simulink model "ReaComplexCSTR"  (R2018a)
settings: Solver=VariableStepAuto  StartTime=0.0  StopTime=10000  RelTol=1e-3
undefined symbols (not defined in the file): e729db96ecb7, f30486205ece, ReaComplexCSTR, sdiscope

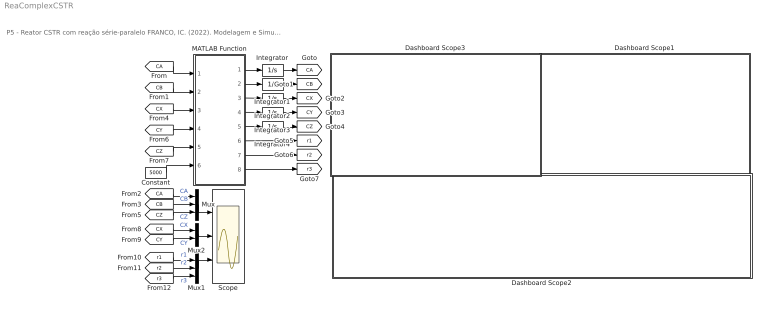
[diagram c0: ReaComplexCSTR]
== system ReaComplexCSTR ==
  note: P5 - Reator CSTR com reação série-paralelo FRANCO, IC. (2022). Modelagem e Simulação: Problemas Típicos da Engenharia Química para Simulação e Análise. NOTAS DE AULA INOVADORAS. The Journal of Engineering and Exact Sciences. Material Complementar.
  Constant : Constant  Value=5000
  Dashboard Scope1 : Subsystem  DialogController=hmiCreateDDGDialog  IsWebBlock=on  mask(MWDashboardBlock){webBlockId=67a52530-171f-4111-9f33-f30486205ece, webBlockType=sdiscope, ShowInitialText=on, HMISrcModelName=ReaComplexCSTR}
      mask prompts: webBlockId "WebBlock Id"; webBlockType "WebBlock Type"; HMISrcModelName "Source Model"
      mask help: SimulinkHMI:dialogs:HMIScopeDialogDesc
  Dashboard Scope2 : Subsystem  DialogController=hmiCreateDDGDialog  IsWebBlock=on  mask(MWDashboardBlock){webBlockId=01cdbba2-3691-40b7-94a4-e729db96ecb7, webBlockType=sdiscope, ShowInitialText=on, HMISrcModelName=ReaComplexCSTR}
      mask prompts: webBlockId "WebBlock Id"; webBlockType "WebBlock Type"; HMISrcModelName "Source Model"
      mask help: SimulinkHMI:dialogs:HMIScopeDialogDesc
  Dashboard Scope3 : Subsystem  DialogController=hmiCreateDDGDialog  IsWebBlock=on  mask(MWDashboardBlock){webBlockId=9a3adbde-0cc4-4c14-8736-21e25775a34c, webBlockType=sdiscope, ShowInitialText=on, HMISrcModelName=ReaComplexCSTR}
      mask prompts: webBlockId "WebBlock Id"; webBlockType "WebBlock Type"; HMISrcModelName "Source Model"
      mask help: SimulinkHMI:dialogs:HMIScopeDialogDesc
  Integrator : Integrator  InitialCondition=0.4
  Integrator1 : Integrator  InitialCondition=0.6
  Integrator2 : Integrator
  Integrator3 : Integrator
  Integrator4 : Integrator
  MATLAB Function : MATLAB Function  TreatAsAtomicUnit=on
  Mux : Mux  Inputs=3
  Mux1 : Mux  Inputs=3
  Mux2 : Mux  Inputs=2
  Scope : Scope  NumInputPorts=3
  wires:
  Integrator1/1 -> [CB]
  MATLAB Function/2(dCB) -> Integrator1/1
  [CB] -> MATLAB Function/2(CB)
  Integrator/1 -> [CA]
  [CA] -> MATLAB Function/1(CA)
  MATLAB Function/1(dCA) -> Integrator/1
  MATLAB Function/3(dCX) -> Integrator2/1
  Integrator2/1 -> [CX]
  MATLAB Function/5(dCZ) -> Integrator4/1
  MATLAB Function/4(dCY) -> Integrator3/1
  Integrator4/1 -> [CZ]
  Integrator3/1 -> [CY]
  MATLAB Function/6(r1) -> [r1]
  MATLAB Function/7(r2) -> [r2]
  MATLAB Function/8(r3) -> [r3]
  Constant/1 -> MATLAB Function/6(tau)
  [CX] -> MATLAB Function/3(CX)
  [CY] -> MATLAB Function/4(CY)
  [CZ] -> MATLAB Function/5(CZ)
  [CA] -> Mux/1  "CA"
  [CB] -> Mux/2  "CB"
  [r1] -> Mux1/1  "r1"
  [r2] -> Mux1/2  "r2"
  [r3] -> Mux1/3  "r3"
  [CX] -> Mux2/1  "CX"
  [CY] -> Mux2/2  "CY"
  Mux2/1 -> Scope/2
  Mux1/1 -> Scope/3
  Mux/1 -> Scope/1
  [CZ] -> Mux/3  "CZ"

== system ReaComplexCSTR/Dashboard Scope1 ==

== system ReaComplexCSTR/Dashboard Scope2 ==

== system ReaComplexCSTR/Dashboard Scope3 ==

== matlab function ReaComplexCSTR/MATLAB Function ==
function [dCA,dCB,dCX,dCY,dCZ,r1,r2,r3] = fcn(CA,CB,CX,CY,CZ,tau)
%% Parâmetros
CA0  = 0.4;
CB0  = 0.6;
CX0  = 0.0;
CY0  = 0.0;
CZ0  = 0.0;
k1   = 0.0005;
k2   = 0.0500;
k3   = 0.0200;

%% Equações auxiliares;
r1 = k1*CA*CB;
r2 = k2*CB*CX;
r3 = k3*CB*CY;

%% Modelo matemático
dCA = (1/tau)*(CA0-CA)-r1;
dCB = (1/tau)*(CB0-CB)-r1-r2-r3;
dCX = (1/tau)*(CX0-CX)+r1-r2;
dCY = (1/tau)*(CY0-CY)+r2-r3;
dCZ = (1/tau)*(CZ0-CZ)+r3;
end
